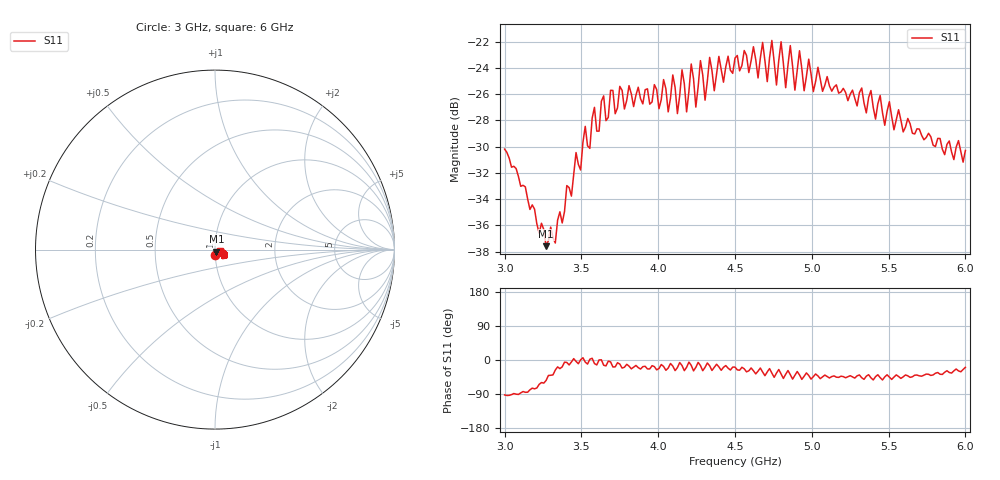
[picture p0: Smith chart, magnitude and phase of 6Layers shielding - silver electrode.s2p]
!  03/07/2025  16:27:09
! Ref Plane: 0.000 mm
# MHZ S MA R  50
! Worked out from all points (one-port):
!   201 points, 3 GHz to 6 GHz, reference 50 ohm
!   lowest |S11| = -37.6 dB at 3.27 GHz (marker M1), VSWR 1.03, Z = 50.8 - j1.09 ohm
!   |S11| at or under -10 dB: start of sweep to end of sweep
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3000  0.03095 -92.2
3270  0.01321 -54.1
3375  0.01619 -18.1
3525  0.03778 -5.5
3555  0.03114 2.0
3585  0.04463 -9.4
3615  0.03622 0.2
3645  0.04936 -13.8
3750  0.05365 -10.7
4005  0.04411 -22.5
4035  0.05694 -17.0
4065  0.0429 -21.3
4095  0.0593 -15.9
4125  0.04227 -20.1
4155  0.06203 -14.4
4185  0.0429 -19.1
4215  0.06529 -14.1
4245  0.04473 -19.4
4275  0.06723 -14.5
4305  0.04753 -19.3
4335  0.06915 -15.3
4365  0.05162 -19.5
4395  0.06979 -18.0
4500  0.06877 -18.7
4875  0.06395 -50.5
5250  0.05008 -41.4
5625  0.04048 -41.7
6000  0.03057 -19.3
